[IBIS VER]   5.0
[File Name]   f28p551pn.ibs
[File Rev]   1.0
[Date]   August 04, 2025
[Source]   File originated at Texas Instruments
[Copyright]   (c) 2012, Texas Instruments Inc.
[Component]   f28p551pn
[Manufacturer]  Texas Instruments
[Package]
| Variable   Typ   Min   Max
R_pkg  1.79E-01  8.06E-02  2.49E-01
L_pkg  6.78E-09  5.42E-09  8.18E-09
C_pkg  6.53E-15  3.76E-15  1.02E-14
[Pin]   signal_name   model_name   R_pin   L_pin   C_pin
   1   GPIO30   BCF3385DSHYPBFZ_LC  2.07E-01  7.68E-09  1.03E-14
   2   GPIO31   BCF3385DSHYPBFZ_LC  1.88E-01  7.34E-09  4.90E-15
   3   GPIO29   BCF3385DSHYPBFZ_LC  1.67E-01  6.98E-09  4.65E-15
   4   A16,B16,C16,GPIO28   BCF3385DSHYPBFZ_LC  1.62E-01  6.79E-09  4.52E-15
   5   XRSn   BQ0491FS_USF  1.56E-01  6.59E-09  4.39E-15
   6   GPIO46   BCF3385DSHYPBFZ_LC  1.53E-01  6.41E-09  4.27E-15
   7   VDDIO   NC  1.59E-01  6.33E-09  4.22E-15
   8   VDD   NC  9.76E-02  5.56E-09  9.16E-15
   9   VSS   NC  9.83E-02  5.42E-09  8.90E-15
   10   A6,D14,E14,GPIO228   BCF3385DSHYPBFZ_LC_USF  1.59E-01  5.90E-09  9.10E-15
   11   B2,C6,E12,GPIO226   BCF3385DSHYPBFZ_LC_USF  1.56E-01  5.87E-09  9.08E-15
   12   A3,B3,C5,GPIO242,PGA2_INP   BCF3385DSHYPBFZ_LC_USF  1.56E-01  6.02E-09  9.35E-15
   13   A2,B6,C9,GPIO224,PGA1_INP   BCF3385DSHYPBFZ_LC  1.55E-01  6.16E-09  9.60E-15
   14   A15,B9,C7,PGA1_INM   ICF33SHYPB_LC  1.54E-01  6.28E-09  4.19E-15
   15   A14,B14,C4,PGA1_OUT   ICF33SHYPB_LC  1.54E-01  6.42E-09  4.28E-15
   16   A11,B10,C0,PGA2_OUT   ICF33SHYPB_LC  1.52E-01  6.55E-09  4.36E-15
   17   A5,B12,C2,PGA2_INM   ICF33SHYPB_LC  1.54E-01  6.71E-09  4.47E-15
   18   A1,B7,D11,DACB_OUT   ICF33SHYPB_LC  1.57E-01  6.89E-09  4.58E-15
   19   A0,B15,C15,DACA_OUT   ICF33SHYPB_LC  1.66E-01  7.12E-09  4.74E-15
   20   D20,E20,VREFHI   ICF33SHYPB_LC  8.43E-02  6.42E-09  4.21E-15
   21   A13,B13,C13,D13,E13,VREFLO   ICF33SHYPB_LC  8.53E-02  6.49E-09  4.25E-15
   22   A12,C1,E11,PGA3_INP   ICF33SHYPB_LC  1.69E-01  7.21E-09  4.80E-15
   23   A7,B30,C3,D12,E30,PGA3_INM   ICF33SHYPB_LC  1.67E-01  7.04E-09  4.69E-15
   24   A8,B0,C11,PGA3_OUT   ICF33SHYPB_LC  1.63E-01  6.86E-09  4.57E-15
   25   VSSA   NC  8.08E-02  5.87E-09  3.85E-15
   26   VDDA   NC  8.06E-02  5.72E-09  3.76E-15
   27   A4,B8,C14   ICF33SHYPB_LC  1.69E-01  6.48E-09  4.33E-15
   28   A9,B4,C8,GPIO227,GPIO236   BCF3385DSHYPBFZ_LC  1.92E-01  6.58E-09  9.97E-15
   29   A10,B1,C10,GPIO230   BCF3385DSHYPBFZ_LC  1.93E-01  6.44E-09  9.71E-15
   30   VSS   NC  1.14E-01  5.49E-09  8.84E-15
   31   GPIO62   BCF3385DSHYPBFZ_LC  2.09E-01  6.46E-09  9.56E-15
   32   GPIO63   BCF3385DSHYPBFZ_LC  1.93E-01  6.44E-09  9.71E-15
   33   A17,B17,C17,CMP1_DACL,GPIO20   BCF3385DSHYPBFZ_LC  1.81E-01  6.47E-09  9.89E-15
   34   A18,B18,C18,GPIO21   BCF3385DSHYPBFZ_LC  1.77E-01  6.57E-09  4.40E-15
   35   A19,B19,C19,GPIO13   BCF3385DSHYPBFZ_LC  1.69E-01  6.63E-09  4.43E-15
   36   A20,B20,C20,GPIO12   BCF3385DSHYPBFZ_LC  1.62E-01  6.71E-09  4.47E-15
   37   A24,D0,E0,GPIO11   BCF3385DSHYPBFZ_LC  1.60E-01  6.82E-09  4.54E-15
   38   B24,D1,E1,GPIO33   BCF3385DSHYPBFZ_LC  1.73E-01  7.10E-09  4.74E-15
   39   C24,D2,E2,GPIO16   BCF3385DSHYPBFZ_LC  1.83E-01  7.35E-09  4.90E-15
   40   A25,D3,E3,GPIO17   BCF3385DSHYPBFZ_LC  1.99E-01  7.65E-09  1.02E-14
   41   B25,D4,E4,GPIO24   BCF3385DSHYPBFZ_LC  2.00E-01  7.61E-09  1.01E-14
   42   GPIO25   BCF3385DSHYPBFZ_LC  1.93E-01  7.40E-09  4.94E-15
   43   GPIO26   BCF3385DSHYPBFZ_LC  1.87E-01  7.19E-09  4.80E-15
   44   GPIO27   BCF3385DSHYPBFZ_LC  1.84E-01  7.02E-09  4.70E-15
   45   TCK   BCF3355DSHYPBFZ_TMS_USF  1.86E-01  6.89E-09  4.61E-15
   46   GPIO37/TDO   BCPF335585DSHYPBFZ  1.84E-01  6.73E-09  4.51E-15
   47   TMS   BCF3355DSHYPBFZ_TMS  1.85E-01  6.60E-09  4.42E-15
   48   GPIO35/TDI   BCF3385DSHYPBFZ_LC  1.88E-01  6.49E-09  9.85E-15
   49   GPIO32   BQ3320HYPBFZ_3VSBLK_5FS_LC  1.91E-01  6.38E-09  9.61E-15
   50   GPIO18,X2   BCF3385DSHYPBFZ_LC  1.87E-01  6.19E-09  9.31E-15
   51   GPIO19,X1   BCPF335585DSHYPBFZ  2.05E-01  6.38E-09  9.45E-15
   52   VDDIO   NC  2.04E-01  6.51E-09  9.71E-15
   53   VDD   NC  1.10E-01  5.69E-09  9.26E-15
   54   GPIO43   BCF3385DSHYPBFZ_LC  1.87E-01  6.62E-09  4.44E-15
   55   VREGENZ,VSS   NC  8.73E-02  5.74E-09  3.77E-15
   56   GPIO39   BCF3385DSHYPBFZ_LC  1.95E-01  7.13E-09  4.77E-15
   57   GPIO42   BCF3385DSHYPBFZ_LC  1.95E-01  7.13E-09  4.77E-15
   58   GPIO8   BCF3385DSHYPBFZ_LC  2.04E-01  7.36E-09  4.93E-15
   59   GPIO4   BCF3385DSHYPBFZ_LC  2.07E-01  7.54E-09  5.05E-15
   60   GPIO3  BQ3320HYPBFZ_3VSBLK_5FS_LC  2.29E-01  7.90E-09  1.06E-14
   61   GPIO2  BQ3320HYPBFZ_3VSBLK_5FS_LC  2.49E-01  8.18E-09  1.10E-14
   62   GPIO1   BCF3385DSHYPBFZ_LC  2.44E-01  7.98E-09  5.37E-15
   63   GPIO0   BCF3385DSHYPBFZ_LC  2.36E-01  7.75E-09  5.21E-15
   64   GPIO40   BCF3385DSHYPBFZ_LC  2.29E-01  7.53E-09  5.07E-15
   65   GPIO23   BCF3385DSHYPBFZ_LC   2.27E-01  7.37E-09  4.96E-15
   66   GPIO41   BCF3385DSHYPBFZ_LC  2.24E-01  7.20E-09  4.85E-15
   67   GPIO22   BCF3385DSHYPBFZ_LC  2.23E-01  7.05E-09  4.75E-15
   68   GPIO7   BCF3385DSHYPBFZ_LC  2.22E-01  6.89E-09  1.02E-14
   69   GPIO44   BCF3385DSHYPBFZ_LC  2.26E-01  6.79E-09  9.96E-15
   70   VSS   NC  1.31E-01  5.67E-09  8.98E-15
   71   VDD   NC  1.40E-01  5.76E-09  9.04E-15
   72   VDDIO   NC  2.37E-01  6.90E-09  1.00E-14
   73   GPIO45   BCF3385DSHYPBFZ_LC  2.22E-01  6.89E-09  1.02E-14
   74   GPIO5   BCF3385DSHYPBFZ_LC  2.22E-01  7.03E-09  4.74E-15
   75   GPIO9  BQ3320HYPBFZ_3VSBLK_5FS_LC  2.20E-01  7.16E-09  4.82E-15
   76   GPIO10   BCF3385DSHYPBFZ_LC_USF  2.21E-01  7.31E-09  4.92E-15
   77   GPIO34   BCF3385DSHYPBFZ_LC_USF  2.19E-01  7.44E-09  4.99E-15
   78   GPIO15   BCF3385DSHYPBFZ_LC_USF  2.19E-01  7.58E-09  5.09E-15
   79   GPIO14   BCF3385DSHYPBFZ_LC_USF  2.21E-01  7.74E-09  5.19E-15
   80   GPIO6   BCF3385DSHYPBFZ_LC_USF  2.27E-01  7.94E-09  1.06E-14
| End of package information
|   Component BQ0491FS_USF
[Component]   BQ0491FS_USF
[Manufacturer]   Texas Instruments
[Package]
|  variable   typ   min   max
R_pkg   0   0   0
L_pkg   0   0   0
C_pkg   0   0   0
[Pin]   signal_name   model_name   R_pin   L_pin   C_pin
VSS   VSS   GND
VDDS   VDDS   POWER
PAD   PAD   BQ0491FS_USF
[Model Selector] BQ0491FS_USF
WK_PU_ON_WITH_RX_3P3  Cell operated at 3.3(nom)
|WK_PU_ON_WITH_RX_3P3; WEAK_PULLUP_ON_WITH_RX
OPEN_DRAIN_MODE_3P3  Cell operated at 3.3(nom)
|   Component BCPF335585DSHYPBFZ
[Component]   BCPF335585DSHYPBFZ
[Manufacturer]   Texas Instruments
[Package]
|  variable   typ   min   max
R_pkg   0   0   0
L_pkg   0   0   0
C_pkg   0   0   0
[Pin]   signal_name   model_name   R_pin   L_pin   C_pin
VSS   VSS   GND
VDDS   VDDS   POWER
PAD   PAD   BCPF335585DSHYPBFZ
[Model Selector] BCPF335585DSHYPBFZ
BCPF_WK_PU_ON_3P3  Cell operated at 3.3(nom)
|BCPF_WK_PU_ON_3P3; WEAK_PULLUP_ON
BCPF_DRIVER_MODE_4MA_3P3  Cell operated at 3.3(nom)
|BCPF_DRIVER_MODE_4MA_3P3
BCPF_DRIVER_MODE_2MA_3P3  Cell operated at 3.3(nom)
|BCPF_DRIVER_MODE_2MA_3P3
BCPF_WK_PD_ON_3P3  Cell operated at 3.3(nom)
|   Component ICF33SHYPB_LC
[Component]   ICF33SHYPB_LC
[Manufacturer]   Texas Instruments
[Package]
|  variable   typ   min   max
R_pkg   0   0   0
L_pkg   0   0   0
C_pkg   0   0   0
[Pin]   signal_name   model_name   R_pin   L_pin   C_pin
VSS   VSS   GND
VDDS   VDDS   POWER
PAD   PAD   ICF33SHYPB_LC
[Model Selector] ICF33SHYPB_LC
ICF_RECEIVER_MODE_3P3  Cell operated at 3.3(nom)
|ICF_RECEIVER_MODE_3P3; RECEIVER_MODE
ICF_WK_PU_ON_3P3  Cell operated at 3.3(nom)
|ICF_WK_PU_ON_3P3; WEAK_PULLUP_ON
ICF_WK_PD_ON_3P3  Cell operated at 3.3(nom)
|   Component BCF3385DSHYPBFZ_LC_USF
[Component]   BCF3385DSHYPBFZ_LC_USF
[Manufacturer]   Texas Instruments
[Package]
|  variable   typ   min   max
R_pkg   0   0   0
L_pkg   0   0   0
C_pkg   0   0   0
[Pin]   signal_name   model_name   R_pin   L_pin   C_pin
VSS   VSS   GND
VDDS   VDDS   POWER
PAD   PAD   BCF3385DSHYPBFZ_LC_USF
[Model Selector] BCF3385DSHYPBFZ_LC_USF
BCF_WK_PU_ON_3P3  Cell operated at 3.3(nom)
|BCF_WK_PU_ON_3P3; WEAK_PULLUP_ON
BCF_WK_PD_ON_3P3  Cell operated at 3.3(nom)
|BCF_WK_PD_ON_3P3; WEAK_PULLDOWN_ON
BCF_DRIVER_MODE_3P3  Cell operated at 3.3(nom)
|BCF_DRIVER_MODE_3P3
BCF_RECEIVER_MODE_3P3  Cell operated at 3.3(nom)
|   Component BCF3355DSHYPBFZ_TMS_USF
[Component]   BCF3355DSHYPBFZ_TMS_USF
[Manufacturer]   Texas Instruments
[Package]
|  variable   typ   min   max
R_pkg   0   0   0
L_pkg   0   0   0
C_pkg   0   0   0
[Pin]   signal_name   model_name   R_pin   L_pin   C_pin
VSS   VSS   GND
VDDS   VDDS   POWER
PAD   PAD   BCF3355DSHYPBFZ_TMS_USF
[Model Selector] BCF3355DSHYPBFZ_TMS_USF
TMS_WK_PU_ON_3P3  Cell operated at 3.3(nom)
|TMS_WK_PU_ON_3P3; WEAK_PULLUP_ON
TMS_DRIVER_3P3  Cell operated at 3.3(nom)
|TMS_DRIVER_3P3
TMS_WK_PD_ON_3P3  Cell operated at 3.3(nom)
|   Component BCF3385DSHYPBFZ_LC
[Component]   BCF3385DSHYPBFZ_LC
[Manufacturer]   Texas Instruments
[Package]
|  variable   typ   min   max
R_pkg   0   0   0
L_pkg   0   0   0
C_pkg   0   0   0
[Pin]   signal_name   model_name   R_pin   L_pin   C_pin
VSS   VSS   GND
VDDS   VDDS   POWER
PAD   PAD   BCF3385DSHYPBFZ_LC
[Model Selector] BCF3385DSHYPBFZ_LC
BCF_WK_PU_ON_3P3  Cell operated at 3.3(nom)
|BCF_WK_PU_ON_3P3; WEAK_PULLUP_ON
BCF_WK_PD_ON_3P3  Cell operated at 3.3(nom)
|BCF_WK_PD_ON_3P3; WEAK_PULLDOWN_ON
BCF_DRIVER_MODE_3P3  Cell operated at 3.3(nom)
|BCF_DRIVER_MODE_3P3
BCF_RECEIVER_MODE_3P3  Cell operated at 3.3(nom)
|BCF_RECEIVER_MODE_3P3; RECEIVER_MODE
|   Component IQ0440FS_VREGENZ_USF
[Component]   IQ0440FS_VREGENZ_USF
[Manufacturer]   Texas Instruments
[Package]
|  variable   typ   min   max
R_pkg   0   0   0
L_pkg   0   0   0
C_pkg   0   0   0
[Pin]   signal_name   model_name   R_pin   L_pin   C_pin
VSS   VSS   GND
VDDS   VDDS   POWER
PAD   PAD   IQ0440FS_VREGENZ_USF
[Model Selector] IQ0440FS_VREGENZ_USF
VREGENZ_WK_PD_ON_3P3  Cell operated at 3.3(nom)
|VREGENZ_WK_PD_ON_3P3; WEAK_PULLDOWN_ON
VREGENZ_WK_PD_OFF_3P3  Cell operated at 3.3(nom)
|   Component BCF3355DSHYPBFZ_TMS
[Component]   BCF3355DSHYPBFZ_TMS
[Manufacturer]   Texas Instruments
[Package]
|  variable   typ   min   max
R_pkg   0   0   0
L_pkg   0   0   0
C_pkg   0   0   0
[Pin]   signal_name   model_name   R_pin   L_pin   C_pin
VSS   VSS   GND
VDDS   VDDS   POWER
PAD   PAD   BCF3355DSHYPBFZ_TMS
[Model Selector] BCF3355DSHYPBFZ_TMS
TMS_WK_PU_ON_3P3  Cell operated at 3.3(nom)
|TMS_WK_PU_ON_3P3; WEAK_PULLUP_ON
TMS_DRIVER_3P3  Cell operated at 3.3(nom)
|TMS_DRIVER_3P3
TMS_WK_PD_ON_3P3  Cell operated at 3.3(nom)
|TMS_WK_PD_ON_3P3; WEAK_PULLDOWN_ON
|   Component BQ3320HYPBFZ_3VSBLK_5FS_LC
[Component] BQ3320HYPBFZ_3VSBLK_5FS_LC
[Manufacturer] Texas Instruments
[Package]
| variable   typ   min   max
R_pkg   0.0   0.0   0.0
L_pkg   0.0H   0.0H   0.0H
C_pkg   0.0F   0.0F   0.0F
[Pin]  signal_name   model_name   R_pin   L_pin   C_pin
PAD   PAD   BQ3320HYPBFZ_3VSBLK_5FS_LC
VDDS   VDDS   Power
VSS   VSS   Gnd
A   A   NC
GZ   GZ   NC
[Model Selector] BQ3320HYPBFZ_3VSBLK_5FS_LC
BQ3320HYPBFZ_3VSBLK_5FS_LC_M0_D0 I/O model with Mode = 0 and Drive = 0
BQ3320HYPBFZ_3VSBLK_5FS_LC_M0_D1 I/O model with Mode = 0 and Drive = 1
BQ3320HYPBFZ_3VSBLK_5FS_LC_M1_D0 I/O model with Mode = 1 and Drive = 0
BQ3320HYPBFZ_3VSBLK_5FS_LC_M1_D1 I/O model with Mode = 1 and Drive = 1
BQ3320HYPBFZ_3VSBLK_5FS_LC_PDON I/O model with Pulldown on PI=0 PSEL=0
BQ3320HYPBFZ_3VSBLK_5FS_LC_PUON I/O model with Pullup on PI=0 PSEL=0
| Models and submodels in the file (24): WK_PU_ON_WITH_RX_3P3 (Input), OPEN_DRAIN_MODE_3P3 (I/O_open_drain), BCPF_WK_PU_ON_3P3 (Input), BCPF_DRIVER_MODE_4MA_3P3 (I/O), BCPF_DRIVER_MODE_2MA_3P3 (I/O), BCPF_WK_PD_ON_3P3 (Input), ICF_RECEIVER_MODE_3P3 (Input), ICF_WK_PU_ON_3P3 (Input), ICF_WK_PD_ON_3P3 (Input), BCF_WK_PU_ON_3P3 (Input), BCF_WK_PD_ON_3P3 (Input), BCF_DRIVER_MODE_3P3 (I/O), BCF_RECEIVER_MODE_3P3 (Input), TMS_WK_PU_ON_3P3 (Input), TMS_DRIVER_3P3 (I/O), TMS_WK_PD_ON_3P3 (Input), VREGENZ_WK_PD_ON_3P3 (Input), VREGENZ_WK_PD_OFF_3P3 (Input), BQ3320HYPBFZ_3VSBLK_5FS_LC_M0_D0 (I/O), BQ3320HYPBFZ_3VSBLK_5FS_LC_M0_D1 (I/O), BQ3320HYPBFZ_3VSBLK_5FS_LC_M1_D0 (I/O), BQ3320HYPBFZ_3VSBLK_5FS_LC_M1_D1 (I/O), BQ3320HYPBFZ_3VSBLK_5FS_LC_PDON (Input), BQ3320HYPBFZ_3VSBLK_5FS_LC_PUON (Input)
